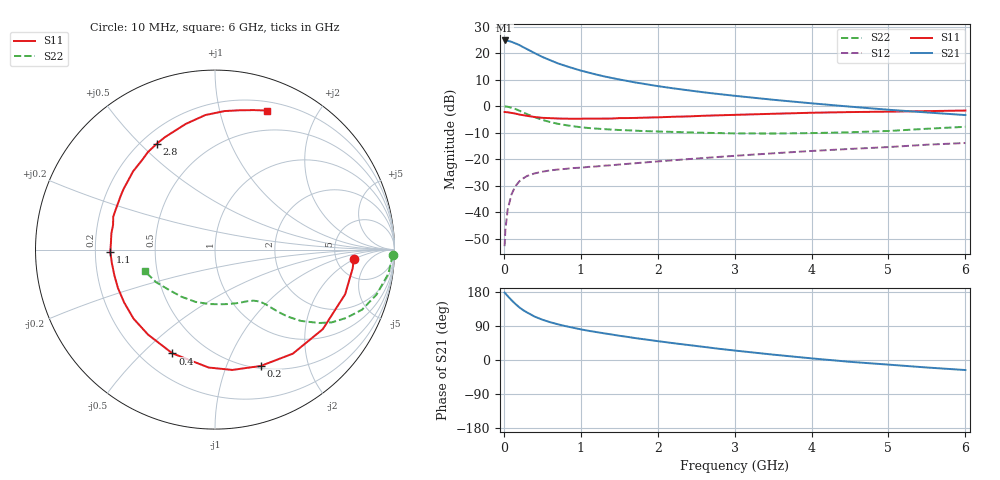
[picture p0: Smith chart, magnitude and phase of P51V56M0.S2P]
! SIEMENS Small Signal Semiconductors
! BFP183
! Si NPN RF Bipolar Junction Transistor in SOT143
! VCE = 1.5 V  IC = 6 mA
! Common Emitter S-Parameters:  March  1996
# GHz  S  MA  R  50
!  f  S11  S21  S12  S22
! GHz  MAG  ANG  MAG  ANG  MAG  ANG  MAG  ANG
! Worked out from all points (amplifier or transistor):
!   36 points, 10 MHz to 6 GHz, reference 50 ohm
!   highest |S21| = 24.8 dB at 10 MHz (marker M1)
!   |S21| within 3 dB of that: start of sweep to 283.5 MHz
!   unconditionally stable (mu >= 1): 1.371 GHz to 5.847 GHz
!   at 250 MHz: K = 0.23, MSG = 24.8 dB, |S12| = -27.3 dB
!   at 1.4 GHz: K = 1.02, MAG = 15.7 dB, |S12| = -22.3 dB
!   at 6 GHz: K = 0.98, MSG = 5.3 dB, |S12| = -13.9 dB
!   S11 on the Smith chart (normalised r, x): 10 MHz: 7.42, -1.86; 200 MHz: 0.53, -1.33; 400 MHz: 0.33, -0.62; 1.1 GHz: 0.26, -0.01; 2.8 GHz: 0.26, +0.56; 6 GHz: 0.29, +1.40
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0.01  0.7752 -3.7  17.31 177.9  0.0023 89.4  0.9901 -1.7
0.02  0.774 -7.8  17.24 175.9  0.0047 86.6  0.986 -3.2
0.05  0.7667 -18.9  17.1 168.7  0.0113 80.7  0.9749 -8.0
0.1  0.7465 -36.4  16.3 157.9  0.0218 71.3  0.934 -15.6
0.15  0.724 -53.2  15.26 148.0  0.031 64.5  0.8853 -22.2
0.2  0.6965 -68.6  14.24 139.1  0.0381 58.3  0.8245 -27.5
0.25  0.6774 -81.8  12.97 131.7  0.0434 52.9  0.7656 -32.0
0.3  0.658 -93.1  11.92 125.7  0.0482 48.2  0.7095 -35.2
0.4  0.625 -112.3  10.01 114.6  0.0541 42.0  0.6219 -39.7
0.5  0.6029 -128.2  8.474 106.4  0.0582 38.0  0.5522 -42.6
0.6  0.595 -139.7  7.378 99.9  0.0616 35.7  0.5025 -44.3
0.7  0.5858 -149.6  6.421 94.4  0.0639 34.2  0.4665 -45.4
0.9  0.5787 -165.7  5.182 85.2  0.0682 32.8  0.419 -47.0
1.1  0.5833 -178.7  4.302 77.1  0.0717 32.1  0.3878 -48.8
1.5  0.5958 162.2  3.187 64.0  0.0795 32.8  0.3556 -53.1
1.8  0.6058 149.7  2.666 55.3  0.0863 33.4  0.3403 -57.6
2.2  0.6311 136.3  2.171 44.5  0.0955 33.6  0.3272 -64.6
2.8  0.6732 118.8  1.689 29.5  0.1107 32.8  0.3108 -77.7
3.5  0.7189 103.1  1.321 14.2  0.1293 30.7  0.3052 -95.7
4.5  0.7738 86.0  0.98 -4.8  0.1564 25.3  0.3223 -125.5
5.5  0.8069 74.4  0.761 -19.8  0.1879 19.7  0.3753 -151.1
6  0.8273 69.5  0.68 -26.5  0.2024 15.5  0.4088 -162.8
